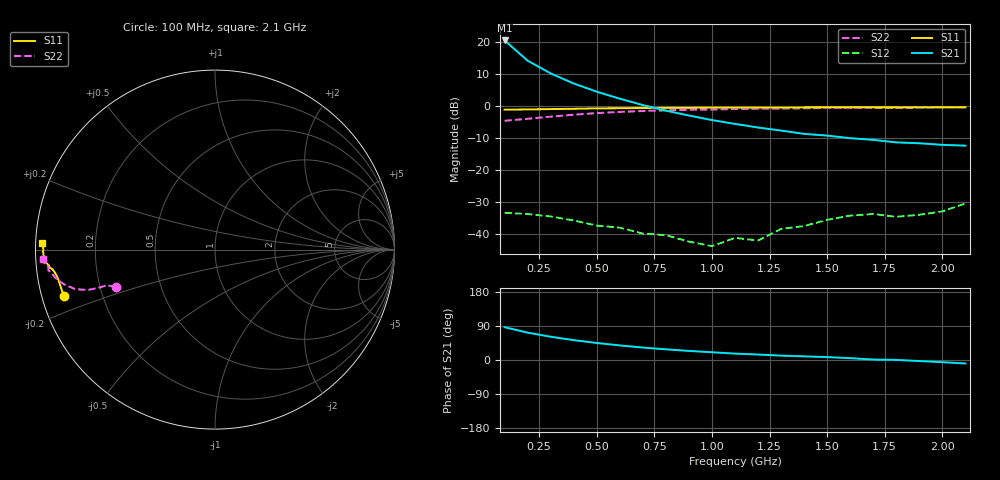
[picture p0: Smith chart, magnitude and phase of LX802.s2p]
! Date: Mon Aug 07 11:24:30 1995
# MHZ  S  MA  R  50.0000
!  POLYFET RF DEVICES
!  LX802 -  L88082
!  S PARAMETERS
!  VDS=28V, IDQ=800mA
! FREQ  S11MAG  S11ANG  S21MAG  S21ANG  S12MAG  S12ANG  S22MAG  S22ANG
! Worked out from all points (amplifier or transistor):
!   21 points, 100 MHz to 2.1 GHz, reference 50 ohm
!   highest |S21| = 20.5 dB at 100 MHz (marker M1)
!   |S21| within 3 dB of that: start of sweep to 147.5 MHz
!   unconditionally stable (mu >= 1): 829.9 MHz to 1.255 GHz
!   at 400 MHz: K = 0.40, MSG = 21.4 dB, |S12| = -35.7 dB
!   at 1.1 GHz: K = 1.10, MAG = 15.9 dB, |S12| = -41.1 dB
!   at 2.1 GHz: K = -0.52, MSG = 9.0 dB, |S12| = -30.4 dB
100  0.881 -162.8  10.63 86.5  0.02164 0.5  0.5913 -159.5
200  0.8905 -169.9  5.141 72.1  0.02068 -11.1  0.6356 -161.8
300  0.901 -171.8  3.247 61.4  0.01895 -16.5  0.6868 -161.9
400  0.9106 -173.0  2.261 52.4  0.01642 -21.4  0.7364 -162.3
500  0.9259 -173.8  1.683 44.9  0.01367 -22.7  0.7793 -163.4
600  0.9293 -174.5  1.309 38.4  0.01266 -21.0  0.8143 -164.5
700  0.9373 -175.1  1.041 32.8  0.01024 -20.2  0.8411 -165.9
800  0.9437 -175.5  0.8518 28.2  0.00967 -11.3  0.8629 -167.0
900  0.9452 -175.7  0.7146 24.0  0.00768 -10.2  0.8789 -168.2
1000  0.9502 -176.3  0.6074 20.5  0.00651 15.9  0.8877 -168.9
1100  0.9524 -176.9  0.5293 16.8  0.00878 26.1  0.9031 -169.9
1200  0.9526 -177.4  0.4643 14.4  0.00798 29.3  0.9112 -171.0
1300  0.9542 -177.9  0.4159 11.5  0.01209 45.7  0.9202 -171.6
1400  0.9564 -178.2  0.3694 9.6  0.01344 48.6  0.9258 -172.3
1500  0.9567 -178.7  0.3472 7.7  0.01675 42.8  0.9357 -173.0
1600  0.9582 -179.4  0.3164 4.9  0.01955 39.3  0.9336 -173.9
1700  0.9565 -179.9  0.2978 1.2  0.02072 34.0  0.9366 -174.3
1800  0.9573 179.6  0.272 0.3  0.01871 31.3  0.944 -174.5
1900  0.959 178.9  0.2638 -2.8  0.02015 28.0  0.955 -175.5
2000  0.9604 178.3  0.249 -5.7  0.02272 25.0  0.9594 -176.4
2100  0.962 178.0  0.2419 -9.2  0.03032 19.8  0.9615 -176.8
